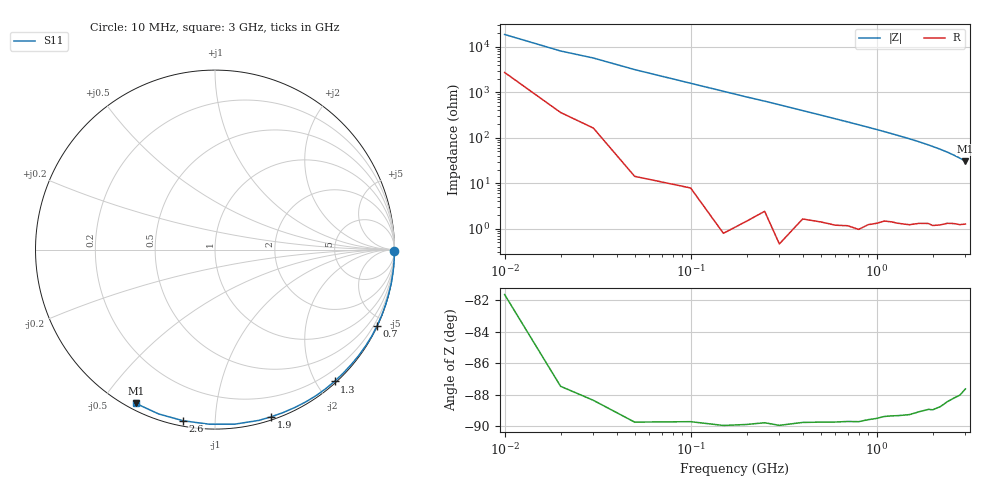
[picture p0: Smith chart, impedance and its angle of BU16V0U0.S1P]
! SIEMENS Small Signal Semiconductors
! BB833
! Si Tuning Diode in SOD323
! VR = 16 V
! S-Parameters:  April  1996
# GHz  S  MA  R  50
!  f  S11
! GHz  MAG  ANG
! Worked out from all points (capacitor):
!   31 points, 10 MHz to 3 GHz, reference 50 ohm
!   read as one part to ground: C = 927 fF near 10 MHz
!   lowest |Z| = 30.5 ohm at 3 GHz (marker M1)
!   S11 on the Smith chart (normalised r, x): 10 MHz: open; 700 MHz: 0.02, -4.47; 1.3 GHz: 0.03, -2.26; 1.9 GHz: 0.03, -1.39; 2.6 GHz: 0.03, -0.83; 3 GHz: 0.03, -0.61
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0.01  0.9992 -0.3
0.05  0.9999 -1.8
0.1  0.9997 -3.6
0.2  0.9998 -7.2
0.25  0.9994 -8.9
0.3  0.9998 -10.7
0.4  0.999 -14.3
0.5  0.9986 -17.9
0.6  0.9983 -21.6
0.7  0.9978 -25.2
0.8  0.9976 -28.9
0.9  0.9962 -32.6
1  0.9949 -36.3
1.1  0.9931 -40.1
1.2  0.9921 -43.9
1.3  0.9914 -47.8
1.4  0.9905 -51.6
1.5  0.9895 -55.4
1.6  0.9877 -59.3
1.7  0.9857 -63.3
1.8  0.9841 -67.4
1.9  0.9825 -71.4
2  0.9826 -75.5
2.2  0.9787 -83.6
2.4  0.9732 -92.0
2.6  0.9699 -100.5
2.8  0.968 -108.9
3  0.9639 -117.3
